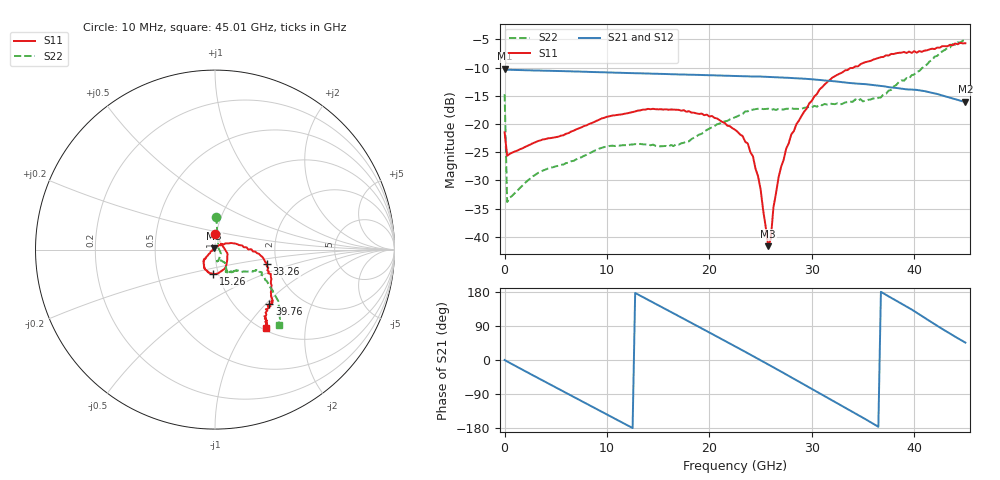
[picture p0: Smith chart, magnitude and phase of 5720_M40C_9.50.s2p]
! Device:  ADRF5720
! Description: 0.5dB LSB GaAs MMIC 6-bit Digital Attenuator
! Frequency:  0.000009 -  40 GHz
! Ports:
!	RF1	= Port 1
!	RF2	= Port 2
! Vdd:  3.3 Volt
! Vss:  -3.3 Volt
! Control:  0/3.3 Volt
! State:  9.50 dB attenuation
! Data:  The device was measured using G-S-G Probes on a matrix board.
!  Data was collected using an calibrated 4 port network analyzer.
!  The reference plane for this measurement is at the launchers.
! Note:  Analog Devices supplies this data as a sample of measured data
!  for this product.  Your particular data for this product may vary.
!  Data was taken at -40 degrees C.
!  Analog Devices reserves the right to change this data at anytime.
# GHZ S DB R 45.0
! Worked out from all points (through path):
!   181 points, 10 MHz to 45.01 GHz, reference 45 ohm
!   highest |S21| = -10.20 dB at 10 MHz (marker M1); lowest = -16.1 dB at 45.01 GHz (marker M2)
!   group delay of S21, straight-line fit = 41.3 ps
!   lowest |S11| = -41.6 dB at 25.76 GHz (marker M3), VSWR 1.02, Z = 44.5 + j0.561 ohm
!   |S11| at or under -10 dB: start of sweep to 34.07 GHz
!   |S22| runs from -33.8 to -5.2 dB; largest |S21 - S12| = 0.0011
!   S11 on the Smith chart (normalised r, x): 10 MHz: 0.99, +0.17; 15.26 GHz: 0.95, -0.26; 33.26 GHz: 1.78, -0.31; 39.76 GHz: 1.42, -1.05; 45.01 GHz: 1.04, -1.24
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0.01  -21.45 88.9  -10.20 -0.1  -10.23 -0.1  -14.71 87.8
0.26  -25.62 7.9  -10.37 -4.0  -10.39 -4.0  -33.83 20.4
4.26  -22.52 -20.2  -10.56 -61.7  -10.58 -61.7  -27.87 -36.4
7.76  -20.36 -45.7  -10.72 -111.8  -10.74 -111.8  -25.64 -62.3
11.51  -18.26 -69.3  -10.93 -165.3  -10.94 -165.4  -23.75 -76.3
15.26  -17.37 -93.8  -11.10 141.0  -11.12 140.9  -23.95 -75.7
19.01  -18.21 -115.1  -11.29 87.0  -11.32 86.9  -21.87 -56.0
22.76  -21.37 -137.5  -11.49 32.5  -11.51 32.4  -18.62 -58.1
24.26  -25.70 -141.0  -11.57 10.6  -11.59 10.4  -17.46 -60.8
25.01  -31.57 -155.7  -11.58 -0.6  -11.61 -0.8  -17.26 -61.0
25.76  -41.65 130.3  -11.65 -11.9  -11.67 -12.0  -17.28 -62.3
26.01  -40.34 90.5  -11.66 -15.6  -11.68 -15.7  -17.48 -63.0
26.26  -34.81 63.5  -11.67 -19.4  -11.69 -19.5  -17.37 -62.0
26.76  -29.49 49.3  -11.73 -26.9  -11.75 -27.1  -17.33 -62.6
27.51  -24.34 29.6  -11.77 -38.2  -11.79 -38.3  -17.29 -63.9
28.51  -20.01 21.6  -11.89 -53.3  -11.91 -53.5  -17.30 -63.7
30.26  -15.10 4.2  -12.10 -80.1  -12.12 -80.3  -16.77 -61.3
33.26  -10.48 -15.4  -12.63 -125.9  -12.66 -126.0  -16.17 -54.0
37.76  -7.57 -40.6  -13.51 164.2  -13.53 164.0  -13.94 -37.2
39.76  -7.38 -44.8  -13.89 133.3  -13.91 133.1  -11.35 -25.1
42.26  -6.44 -53.4  -14.67 90.2  -14.70 90.0  -7.91 -36.3
45.01  -5.67 -57.0  -16.06 45.9  -16.09 45.7  -5.18 -49.7
